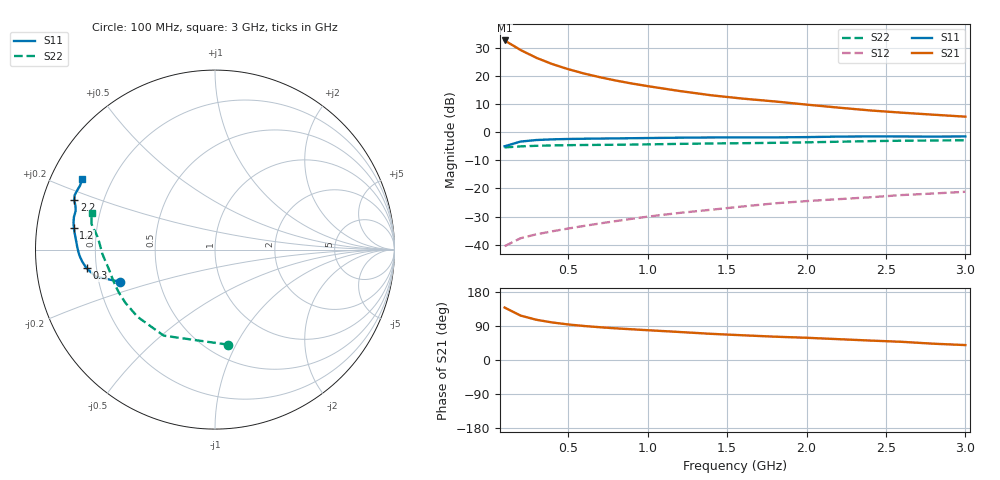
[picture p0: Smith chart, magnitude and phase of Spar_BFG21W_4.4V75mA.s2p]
! Filename: 4_475bfg21.001
! Title: BFG21W
! Bias: Vce=4.4V; Ic=75mA
! Company: NXP Semiconductors NL
! User: Quality&Reliability T&D
! Measure time: 10 Nov 1999 / 11:46:49
#  MHz  S  MA  R 50
! Freq  S11  S21  S12  S22  :
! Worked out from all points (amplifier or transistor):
!   20 points, 100 MHz to 3 GHz, reference 50 ohm
!   highest |S21| = 32.5 dB at 100 MHz (marker M1)
!   |S21| within 3 dB of that: start of sweep to 189.2 MHz
!   unconditionally stable (mu >= 1): 704.7 MHz to end of sweep
!   at 400 MHz: K = 0.84, MSG = 29.7 dB, |S12| = -35.2 dB
!   at 1.2 GHz: K = 1.08, MAG = 20.0 dB, |S12| = -28.7 dB
!   at 3 GHz: K = 1.05, MAG = 11.9 dB, |S12| = -21.2 dB
!   S11 on the Smith chart (normalised r, x): 100 MHz: 0.29, -0.15; 300 MHz: 0.16, -0.07; 1.2 GHz: 0.11, +0.07; 2.2 GHz: 0.09, +0.17; 3 GHz: 0.09, +0.25
100  0.5603 -161.4  42.17 138.4  0.009483 44.4  0.5349 -82.1
200  0.679 -167.1  28.63 117.3  0.01311 43.7  0.5582 -120.8
300  0.7233 -171.7  20.75 106.2  0.01539 46.2  0.5714 -139.0
400  0.7431 -174.9  16.08 99.1  0.0174 49.9  0.5806 -149.2
500  0.755 -177.3  13.06 93.8  0.0195 53.2  0.5865 -155.7
600  0.7625 -179.4  10.93 89.7  0.02168 56.2  0.5904 -160.3
700  0.7681 178.8  9.398 86.4  0.02399 59.1  0.5933 -163.8
800  0.7731 177.0  8.207 83.5  0.02641 61.4  0.5964 -166.7
900  0.7786 175.5  7.275 81.1  0.02895 63.6  0.6007 -169.2
1000  0.7845 174.0  6.532 78.6  0.03168 65.0  0.6058 -171.4
1200  0.7955 171.3  5.358 73.9  0.03684 67.1  0.6178 -175.1
1400  0.8027 169.2  4.497 69.0  0.04199 68.4  0.6287 -178.0
1600  0.8067 166.9  3.919 65.2  0.04801 69.5  0.6357 179.4
1800  0.8056 164.5  3.497 61.6  0.05453 70.1  0.6449 176.7
2000  0.815 162.6  3.071 58.7  0.05975 71.1  0.658 173.9
2200  0.8316 160.6  2.719 55.0  0.06464 71.2  0.6745 171.5
2400  0.8386 158.8  2.421 51.3  0.06981 70.7  0.6915 169.8
2600  0.836 156.9  2.21 48.0  0.07649 69.9  0.7029 168.2
2800  0.8323 154.6  2.033 43.0  0.08149 68.4  0.7088 166.1
3000  0.8374 152.1  1.877 39.4  0.08742 67.6  0.7172 163.6
